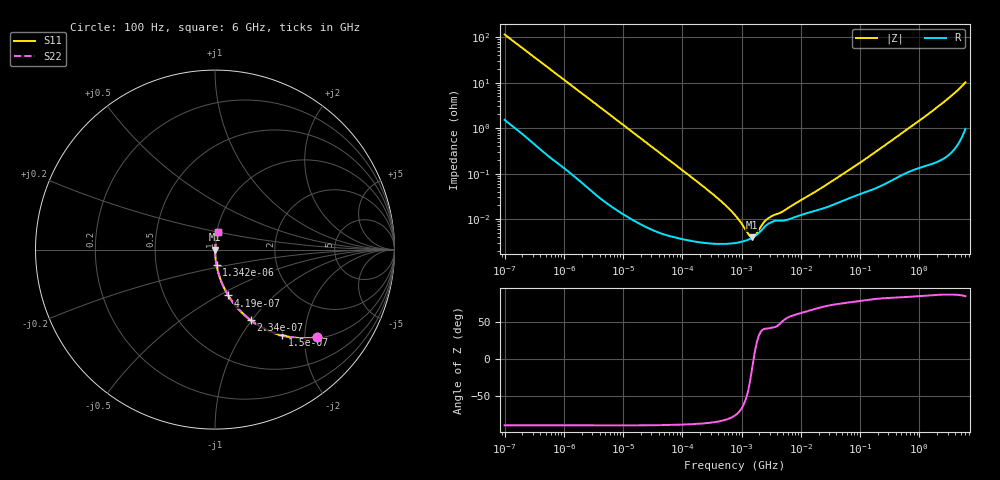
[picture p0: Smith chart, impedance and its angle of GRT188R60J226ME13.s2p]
!Murata Part Number: GRT188R60J226ME13
!These Parameters are Measured in Series Mode Connection
!Data Generated on Jun 19, 2026
!  o--ll--o
!Port1  Port2
!  o------o
!Operation Temp=25[degC], DC Bias Voltage=0[V]
!Freq. Start=100[Hz] Stop=6[GHz] 401[Steps]
# Hz S RI R 50
!Freq.(Hz) S11(Real) S11(Imag) S21(Real) S21(Imag) S12(Real) S12(Imag) S22(Real) S22(Imag)
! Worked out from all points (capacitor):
!   401 points, 100 Hz to 6 GHz, reference 50 ohm
!   read as one part in series: C = 13.8 uF near 109 Hz
!   lowest |Z| = 3.97 mohm at 1.516 MHz (marker M1)
!   series resonance near 1.598 MHz, so ESL is about 720 pH
!   S11 on the Smith chart (normalised r, x): 100 Hz: 1.03, -2.29; 150 Hz: 1.02, -1.54; 234 Hz: 1.01, -0.99; 419 Hz: 1.01, -0.55; 1.342 kHz: 1.00, -0.17; 6 GHz: 1.02, +0.20
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100  0.567 -0.4889  0.433 0.4889  0.433 0.4889  0.567 -0.4889
150  0.3731 -0.4772  0.6269 0.4772  0.6269 0.4772  0.3731 -0.4772
234  0.1987 -0.3927  0.8013 0.3927  0.8013 0.3927  0.1987 -0.3927
419  0.0737 -0.2556  0.9263 0.2556  0.9263 0.2556  0.0737 -0.2556
717  0.0274 -0.1576  0.9726 0.1576  0.9726 0.1576  0.0274 -0.1576
1342  0.00849 -0.0863  0.9915 0.0863  0.9915 0.0863  0.00849 -0.0863
2008  0.00402 -0.0581  0.996 0.0581  0.996 0.0581  0.00402 -0.0581
6433  0.000523 -0.0183  0.9995 0.0183  0.9995 0.0183  0.000523 -0.0183
40335  5.91e-05 -0.00295  0.9999 0.00295  0.9999 0.00295  5.91e-05 -0.00295
330837  2.89e-05 -0.000349  1 0.000349  1 0.000349  2.89e-05 -0.000349
541393  2.87e-05 -0.000197  1 0.000197  1 0.000197  2.87e-05 -0.000197
774597  2.98e-05 -0.000119  1 0.000119  1 0.000119  2.98e-05 -0.000119
926525  3.1e-05 -8.64e-05  1 8.64e-05  1 8.64e-05  3.1e-05 -8.64e-05
1516199  3.89e-05 -7.8e-06  1 7.8e-06  1 7.8e-06  3.89e-05 -7.8e-06
2713602  7.62e-05 6.61e-05  0.9999 -6.61e-05  0.9999 -6.61e-05  7.62e-05 6.61e-05
4856642  9.25e-05 0.000112  0.9999 -0.000112  0.9999 -0.000112  9.25e-05 0.000112
1.555665e7  0.000146 0.000333  0.9999 -0.000333  0.9999 -0.000333  0.000146 0.000333
8.527865e7  0.000331 0.00148  0.9997 -0.00148  0.9997 -0.00148  0.000331 0.00148
3.124326e8  0.000688 0.00489  0.9993 -0.00489  0.9993 -0.00489  0.000688 0.00489
1.873145e9  0.00246 0.0267  0.9975 -0.0267  0.9975 -0.0267  0.00246 0.0267
3.505958e9  0.00557 0.0513  0.9944 -0.0513  0.9944 -0.0513  0.00557 0.0513
6e9  0.0195 0.0984  0.9805 -0.0984  0.9805 -0.0984  0.0195 0.0984
